[IBIS Ver]   4.1
[File Name]   sprm794.ibs
[File Rev]   1.0
[Date]   October 17, 2021
[Source]   File originated at Texas Instruments
[Copyright]   (c) 2012, Texas Instruments Inc.
[Component]   f771860xpt
[Manufacturer] Texas Instruments
[Package]
| Variable   Typ   Min   Max
R_pkg   0.124   0.049   0.212
L_pkg   2.96E-9   2.58E-09   4.16E-09
C_pkg   2.89E-13   2.18E-13   3.84E-13
[Pin]   signal_name   model_name   R_pin   L_pin   C_pin
1   GPIO29   BCPF335585DSHYPBFZ   1.27E-01   2.91E-09   2.2748E-13
2   GPIO28   BCF3385DSHYPBFZ_USF   1.19E-01   2.76E-09   2.7043E-13
3   XRSN   BQ0491FS_USF   1.18E-01   2.70E-09   2.5861E-13
4   A6/B2/C6   ICF33SHYPB_USF   1.70E-01   3.38E-09   3.105E-13
5   A3/B3/VDAC,C5   ICF33SHYPB_USF   1.50E-01   3.12E-09   3.4851E-13
6   A2/B6/C9   ICF33SHYPB_USF   1.43E-01   2.95E-09   2.7043E-13
7   A15/B9/C7   ICF33SHYPB_USF   1.32E-01   2.79E-09   2.7364E-13
8   A11/B10/C0   ICF33SHYPB_USF   1.26E-01   2.73E-09   2.543E-13
9   A5/B12/C2   ICF33SHYPB_USF   1.20E-01   2.70E-09   2.876E-13
10   A1/B7/DACB_OUT   ICF33SHYPB_USF   1.18E-01   2.75E-09   2.7509E-13
11   A0/B15/C15/DACA_OUT   ICF33SHYPB_USF   1.33E-01   2.98E-09   2.8767E-13
12   VREFHI   NC   4.93E-02   2.66E-09   2.7937E-13
13   VREFLO   NC   5.12E-02   2.71E-09   2.8484E-13
14   A12,C1   ICF33SHYPB_USF   1.47E-01   3.21E-09   3.1728E-13
15   A7/C3   ICF33SHYPB_USF   1.46E-01   3.15E-09   2.8228E-13
16   A8/B0/C11   ICF33SHYPB_USF   1.49E-01   3.13E-09   3.1572E-13
17   VSSA   NC   5.38E-02   2.63E-09   3.4579E-13
18   VDDA   NC   5.61E-02   2.70E-09   3.3427E-13
19   A4/B8/C14   ICF33SHYPB_USF   1.69E-01   3.38E-09   3.0852E-13
20   A9/B4/C8   ICF33SHYPB_USF   1.75E-01   3.51E-09   3.3237E-13
21   A10/B1/C10   ICF33SHYPB_USF   1.92E-01   3.77E-09   3.0651E-13
22   VSS   NC   9.19E-02   3.21E-09   3.5013E-13
23   VDD   NC   1.00E-01   3.46E-09   3.8395E-13
24   VDDIO   NC   2.12E-01   4.16E-09   3.3035E-13
25   GPIO33   BCPF335585DSHYPBFZ   1.39E-01   3.10E-09   2.348E-13
26   GPIO16   BCF3385DSHYPBFZ   1.28E-01   2.91E-09   2.715E-13
27   GPIO24   BCF3385DSHYPBFZ   1.27E-01   2.85E-09   2.5996E-13
28   TCK   BCF3355DSHYPBFZ_TMS_USF   1.33E-01   2.90E-09   2.5947E-13
29   GPIO37/TDO   BCPF335585DSHYPBFZ   1.27E-01   2.79E-09   2.539E-13
30   TMS   BCF3355DSHYPBFZ_TMS_USF   1.27E-01   2.76E-09   2.4257E-13
31   GPIO35/TDI   BCF3385DSHYPBFZ   1.32E-01   2.82E-09   2.4663E-13
32   GPIO32   BCPF335585DSHYPBFZ   1.41E-01   2.97E-09   2.5741E-13
33   GPIO18/X2   BCPF335585DSHYPBFZ   1.34E-01   2.95E-09   2.9507E-13
34   GPIO19/X1   BCF3385DSHYPBFZ   1.41E-01   3.10E-09   3.3475E-13
35   VDDIO   NC   1.50E-01   2.95E-09   3.7752E-13
36   VDD   NC   7.82E-02   3.04E-09   3.3895E-13
37   VSS   NC   7.58E-02   2.94E-09   2.8573E-13
38   GPIO4   BCF3385DSHYPBFZ_USF   1.10E-01   2.62E-09   2.6415E-13
39   GPIO3   BCF3385DSHYPBFZ_USF   1.13E-01   2.60E-09   2.5577E-13
40   GPIO2   BCF3385DSHYPBFZ   1.18E-01   2.66E-09   2.5542E-13
41   GPIO1   BCPF335585DSHYPBFZ   1.28E-01   2.74E-09   2.6202E-13
42   GPIO0   BCF3385DSHYPBFZ   1.44E-01   2.93E-09   2.513E-13
43   GPIO7   BCF3385DSHYPBFZ_USF   1.26E-01   2.71E-09   2.3674E-13
44   VSS   NC   6.68E-02   2.94E-09   3.088E-13
45   VDD   NC   6.72E-02   2.58E-09   3.2797E-13
46   VDDIO   NC   1.50E-01   3.09E-09   3.0141E-13
47   GPIO5   BCF3385DSHYPBFZ_USF   1.47E-01   3.16E-09   2.8369E-13
48   GPIO6   BCF3385DSHYPBFZ_USF   1.16E-01   2.74E-09   2.1821E-13
| End of package information
|   Component IQ0440FS_VREGENZ_USF
[Component]   IQ0440FS_VREGENZ_USF
[Manufacturer]   Texas Instruments
[Package]
|  variable   typ   min   max
R_pkg   0   0   0
L_pkg   0   0   0
C_pkg   0   0   0
[Pin]   signal_name   model_name   R_pin   L_pin   C_pin
VSS   VSS   GND
VDDS   VDDS   POWER
PAD   PAD   IQ0440FS_VREGENZ_USF
[Model Selector] IQ0440FS_VREGENZ_USF
VREGENZ_WK_PD_ON_3P3  Cell operated at 3.3(nom)
|VREGENZ_WK_PD_ON_3P3; WEAK_PULLDOWN_ON
VREGENZ_WK_PD_OFF_3P3  Cell operated at 3.3(nom)
|   Component ICF33SHYPB_USF
[Component]   ICF33SHYPB_USF
[Manufacturer]   Texas Instruments
[Package]
|  variable   typ   min   max
R_pkg   0   0   0
L_pkg   0   0   0
C_pkg   0   0   0
[Pin]   signal_name   model_name   R_pin   L_pin   C_pin
VSS   VSS   GND
VDDS   VDDS   POWER
PAD   PAD   ICF33SHYPB_USF
[Model Selector] ICF33SHYPB_USF
ICF_WK_PUPD_OFF_3P3  Cell operated at 3.3(nom)
|ICF_WK_PUPD_OFF_3P3; WEAK_PULL_OFF
ICF_WK_PU_ON_3P3  Cell operated at 3.3(nom)
|ICF_WK_PU_ON_3P3; WEAK_PULLUP_ON
ICF_WK_PD_ON_3P3  Cell operated at 3.3(nom)
|   Component ICF33SHYPB_FS_SFII_CUS
[Component]   ICF33SHYPB_FS_SFII_CUS
[Manufacturer]   Texas Instruments
[Package]
|  variable   typ   min   max
R_pkg   0   0   0
L_pkg   0   0   0
C_pkg   0   0   0
[Pin]   signal_name   model_name   R_pin   L_pin   C_pin
VSS   VSS   GND
VDDS   VDDS   POWER
PAD   PAD   ICF33SHYPB_FS_SFII_CUS
[Model Selector] ICF33SHYPB_FS_SFII_CUS
CUS_WK_PUPD_OFF_3P3  Cell operated at 3.3(nom)
|CUS_WK_PUPD_OFF_3P3; WEAK_PULL_OFF
CUS_WK_PU_ON_3P3  Cell operated at 3.3(nom)
|CUS_WK_PU_ON_3P3; WEAK_PULLUP_ON
CUS_WK_PD_ON_3P3  Cell operated at 3.3(nom)
|   Component BT3308BT5FSHYPB_SFII
[Component]   BT3308BT5FSHYPB_SFII
[Manufacturer]   Texas Instruments
[Package]
|  variable   typ   min   max
R_pkg   0   0   0
L_pkg   0   0   0
C_pkg   0   0   0
[Pin]   signal_name   model_name   R_pin   L_pin   C_pin
VSS   VSS   GND
VDDS   VDDS   POWER
PAD   PAD   BT3308BT5FSHYPB_SFII
[Model Selector] BT3308BT5FSHYPB_SFII
BT_OPEN_DRAIN_6MA_3P3  Cell operated at 3.3(nom)
|BT_OPEN_DRAIN_6MA_3P3
BT_WEAK_PD_ON_3P3  Cell operated at 3.3(nom)
|BT_WEAK_PD_ON_3P3
BT_OPEN_DRAIN_3MA_3P3  Cell operated at 3.3(nom)
|BT_OPEN_DRAIN_3MA_3P3
BT_DRIVER_MODE_6MA_3P3  Cell operated at 3.3(nom)
|BT_DRIVER_MODE_6MA_3P3
BT_DRIVER_MODE_3MA_3P3  Cell operated at 3.3(nom)
|BT_DRIVER_MODE_3MA_3P3
BT_WEAK_PU_ON_3P3  Cell operated at 3.3(nom)
|   Component BQ0491FS_USF
[Component]   BQ0491FS_USF
[Manufacturer]   Texas Instruments
[Package]
|  variable   typ   min   max
R_pkg   0   0   0
L_pkg   0   0   0
C_pkg   0   0   0
[Pin]   signal_name   model_name   R_pin   L_pin   C_pin
VSS   VSS   GND
VDDS   VDDS   POWER
PAD   PAD   BQ0491FS_USF
[Model Selector] BQ0491FS_USF
XRSN_WK_PU_ON_3P3  Cell operated at 3.3(nom)
|XRSN_WK_PU_ON_3P3; WEAK_PULLUP_ON
XRSN_OPEN_DRAIN  Cell operated at 3.3(nom)
|   Component BCPF335585DSHYPBFZ
[Component]   BCPF335585DSHYPBFZ
[Manufacturer]   Texas Instruments
[Package]
|  variable   typ   min   max
R_pkg   0   0   0
L_pkg   0   0   0
C_pkg   0   0   0
[Pin]   signal_name   model_name   R_pin   L_pin   C_pin
VSS   VSS   GND
VDDS   VDDS   POWER
PAD   PAD   BCPF335585DSHYPBFZ
[Model Selector] BCPF335585DSHYPBFZ
BCPF_WK_PU_ON_3P3  Cell operated at 3.3(nom)
|BCPF_WK_PU_ON_3P3; WEAK_PULLUP_ON
BCPF_DRIVER_4MA_3P3  Cell operated at 3.3(nom)
|BCPF_DRIVER_4MA_3P3
BCPF_DRIVER_2MA_3P3  Cell operated at 3.3(nom)
|BCPF_DRIVER_2MA_3P3
BCPF_WK_PD_ON_3P3  Cell operated at 3.3(nom)
|   Component BCF3385DSHYPBFZ_USF
[Component]   BCF3385DSHYPBFZ_USF
[Manufacturer]   Texas Instruments
[Package]
|  variable   typ   min   max
R_pkg   0   0   0
L_pkg   0   0   0
C_pkg   0   0   0
[Pin]   signal_name   model_name   R_pin   L_pin   C_pin
VSS   VSS   GND
VDDS   VDDS   POWER
PAD   PAD   BCF3385DSHYPBFZ_USF
[Model Selector] BCF3385DSHYPBFZ_USF
BCF3385DUSF_WK_PU  Cell operated at 3.3(nom)
| BCF3385DUSF_WK_PU; WEAK_PULLUP_ON
BCF3385DUSF_DRIVER_3P3  Cell operated at 3.3(nom)
|BCF3385DUSF_DRIVER_3P3
BCF3385DUSF_WK_PD  Cell operated at 3.3(nom)
|   Component BCF3385DSHYPBFZ
[Component]   BCF3385DSHYPBFZ
[Manufacturer]   Texas Instruments
[Package]
|  variable   typ   min   max
R_pkg   0   0   0
L_pkg   0   0   0
C_pkg   0   0   0
[Pin]   signal_name   model_name   R_pin   L_pin   C_pin
VSS   VSS   GND
VDDS   VDDS   POWER
PAD   PAD   BCF3385DSHYPBFZ
[Model Selector] BCF3385DSHYPBFZ
BCF3385D_WK_PU_3P3  Cell operated at 3.3(nom)
|BCF3385D_WK_PU_3P3; WEAK_PULLUP_ON
BCF3385D_DRIVER_3P3  Cell operated at 3.3(nom)
|BCF3385D_DRIVER_3P3
BCF3385D_WK_PD_3P3  Cell operated at 3.3(nom)
|   Component BCF3355DSHYPBFZ_TMS_USF
[Component]   BCF3355DSHYPBFZ_TMS_USF
[Manufacturer]   Texas Instruments
[Package]
|  variable   typ   min   max
R_pkg   0   0   0
L_pkg   0   0   0
C_pkg   0   0   0
[Pin]   signal_name   model_name   R_pin   L_pin   C_pin
VSS   VSS   GND
VDDS   VDDS   POWER
PAD   PAD   BCF3355DSHYPBFZ_TMS_USF
[Model Selector] BCF3355DSHYPBFZ_TMS_USF
TMS_WK_PU_ON_3P3  Cell operated at 3.3(nom)
|TMS_WK_PU_ON_3P3; WEAK_PULLUP_ON
TMS_DRIVER_3P3  Cell operated at 3.3(nom)
|TMS_DRIVER_3P3
TMS_WK_PD_ON_3P3  Cell operated at 3.3(nom)
|   Component BCF3335DSHYPBFZ
[Component]   BCF3335DSHYPBFZ
[Manufacturer]   Texas Instruments
[Package]
|  variable   typ   min   max
R_pkg   0   0   0
L_pkg   0   0   0
C_pkg   0   0   0
[Pin]   signal_name   model_name   R_pin   L_pin   C_pin
VSS   VSS   GND
VDDS   VDDS   POWER
PAD   PAD   BCF3335DSHYPBFZ
[Model Selector] BCF3335DSHYPBFZ
BCF3335D_WK_PU_3P3  Cell operated at 3.3(nom)
|BCF3335D_WK_PU_3P3; WEAK_PULLUP_ON
BCF3335D_DRIVER_3P3  Cell operated at 3.3(nom)
|BCF3335D_DRIVER_3P3
BCF3335D_WK_PD_3P3  Cell operated at 3.3(nom)
| Models and submodels in the file (32): VREGENZ_WK_PD_ON_3P3 (Input), VREGENZ_WK_PD_OFF_3P3 (Input), ICF_WK_PUPD_OFF_3P3 (Input), ICF_WK_PU_ON_3P3 (Input), ICF_WK_PD_ON_3P3 (Input), CUS_WK_PUPD_OFF_3P3 (Input), CUS_WK_PU_ON_3P3 (Input), CUS_WK_PD_ON_3P3 (Input), BT_OPEN_DRAIN_6MA_3P3 (I/O_open_drain), BT_WEAK_PD_ON_3P3 (Input), BT_OPEN_DRAIN_3MA_3P3 (I/O_open_drain), BT_DRIVER_MODE_6MA_3P3 (I/O), BT_DRIVER_MODE_3MA_3P3 (I/O), BT_WEAK_PU_ON_3P3 (Input), XRSN_WK_PU_ON_3P3 (Input), XRSN_OPEN_DRAIN (I/O_open_drain), BCPF_WK_PU_ON_3P3 (Input), BCPF_DRIVER_4MA_3P3 (I/O), BCPF_DRIVER_2MA_3P3 (I/O), BCPF_WK_PD_ON_3P3 (Input), BCF3385DUSF_WK_PU (Input), BCF3385DUSF_DRIVER_3P3 (I/O), BCF3385DUSF_WK_PD (Input), BCF3385D_WK_PU_3P3 (Input), BCF3385D_DRIVER_3P3 (I/O), BCF3385D_WK_PD_3P3 (Input), TMS_WK_PU_ON_3P3 (Input), TMS_DRIVER_3P3 (I/O), TMS_WK_PD_ON_3P3 (Input), BCF3335D_WK_PU_3P3 (Input), BCF3335D_DRIVER_3P3 (I/O), BCF3335D_WK_PD_3P3 (Input)
